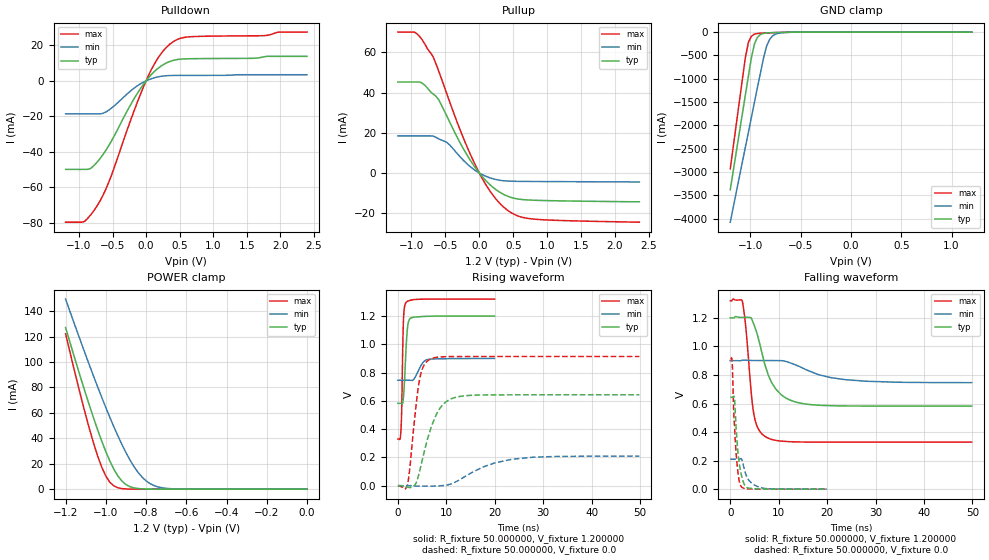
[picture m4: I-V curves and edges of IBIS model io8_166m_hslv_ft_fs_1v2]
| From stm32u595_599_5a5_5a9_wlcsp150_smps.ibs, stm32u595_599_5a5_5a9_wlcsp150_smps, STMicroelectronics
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|   Model io8_166m_hslv_ft_fs_1v2
[Model]  io8_166m_hslv_ft_fs_1v2
Model_type I/O
Polarity   Non-Inverting
Enable   Active-Low
Vinl =   0.360000V
Vinh =   0.840000V
Vmeas =  0.600000V
Cref =   50.000000pF
Rref =   100.000000M
Vref =   0.0V
C_comp   3.151700pF   3.087200pF   3.197900pF
[Temperature Range]   25.000000   0.140000k   -40.000000
[Pullup Reference]   1.200000V   0.900000V   1.320000V
[Pulldown Reference]   0.0V   0.0V   0.0V
[POWER Clamp Reference]   1.200000V   0.900000V   1.320000V
[GND Clamp Reference]   0.0V   0.0V   0.0V
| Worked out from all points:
|   slope of the pulldown table from 0 to 0.18 V, typ, clamps not added: 25.4 ohm
|   slope of the pullup table from 0 to 0.18 V, typ, clamps not added: 27.8 ohm
|   GND clamp passes 1 mA (typ) near -0.51 V on its own axis
|   POWER clamp passes 1 mA (typ) near -0.86 V on its own axis
|   rising waveform, R_fixture 50.000000, V_fixture 1.200000: 20-80 % time 569ps typ, 1.42ns min, 326ps max; typ from 0.582 V to 1.2 V
|   rising waveform, R_fixture 50.000000, V_fixture 0.0: 20-80 % time 3.44ns typ, 8.15ns min, 1.74ns max; typ from 0 V to 0.643 V
|   falling waveform, R_fixture 50.000000, V_fixture 1.200000: 20-80 % time 3.68ns typ, 8.13ns min, 1.62ns max; typ from 1.2 V to 0.582 V
|   falling waveform, R_fixture 50.000000, V_fixture 0.0: 20-80 % time 1.04ns typ, 1.73ns min, 833ps max; typ from 0.643 V to 0 V
[Pulldown]
|Voltage   I(typ)   I(min)   I(max)
-1.2V     -49.86mA   -18.57mA   -79.57mA
-920mV    -49.86mA   -18.57mA   -79.2mA
-840mV    -49.6mA    -18.57mA   -76.08mA
-720mV    -45.32mA   -18.57mA   -69.74mA
-560mV    -36.71mA   -16.58mA   -57.44mA
-200mV    -11.43mA   -4.74mA    -19.03mA
0V        10fA       -600fA     0A
160mV     6.477mA    2.075mA    11.78mA
360mV     10.99mA    2.99mA     20.81mA
480mV     12.07mA    3.054mA    23.53mA
640mV     12.43mA    3.075mA    24.76mA
2.4V      13.79mA    3.434mA    27.44mA
[Pullup]
|Voltage   I(typ)   I(min)   I(max)
-1.2V     45.31mA    18.46mA    70.13mA
-920mV    45.31mA    18.46mA    69.35mA
-840mV    44.69mA    18.46mA    66.15mA
-680mV    39.3mA     18.37mA    57.86mA
-600mV    36.53mA    16.99mA    50.82mA
-480mV    28.42mA    15.27mA    39.5mA
-280mV    14.84mA    7.944mA    21.22mA
-80mV     3.667mA    1.75mA     5.47mA
160mV     -5.889mA   -2.43mA    -9.115mA
400mV     -11.31mA   -3.958mA   -18.11mA
800mV     -13.54mA   -4.214mA   -22.92mA
2.36V     -14.3mA    -4.5mA     -24.47mA
[GND_clamp]
|Voltage   I(typ)   I(min)   I(max)
-1.2V     -3.379A    -4.076A    -2.932A
-1.05V    -1.35A     -2.47A     -550.7mA
-1.02V    -947.8mA   -2.149A    -221.5mA
-990mV    -552.4mA   -1.829A    -88.44mA
-960mV    -255.3mA   -1.51A     -44.87mA
-930mV    -111.8mA   -1.191A    -30.68mA
-870mV    -28.36mA   -564.6mA   -21.34mA
-840mV    -18.65mA   -309.5mA   -18.49mA
-810mV    -14.07mA   -161.6mA   -15.92mA
-780mV    -11.37mA   -83.33mA   -13.53mA
-600mV    -3.009mA   -4.322mA   -3.091mA
1.2V      0A         13.65nA    0A
[POWER_clamp]
|Voltage   I(typ)   I(min)   I(max)
-1.2V     127mA      149.4mA    122.2mA
-1.12V    84.97mA    114mA      70.27mA
-1.06V    55.51mA    88.42mA    35.67mA
-1.02V    37.63mA    72.04mA    17.17mA
-1V       29.51mA    64.13mA    10.3mA
-960mV    15.69mA    48.99mA    2.571mA
-900mV    3.624mA    28.77mA    182.8uA
-840mV    490.7uA    13.24mA    11.35uA
-800mV    116.8uA    6.532mA    1.77uA
-740mV    13.2uA     1.723mA    109.1nA
-620mV    167.4nA    79.36uA    0A
0V        0A         17.87nA    0A
[Ramp]
| variable   typ   min   max
dV/dt_r  0.38561/3.43218n   0.12545/8.14393n   0.54824/1.73724n
dV/dt_f  0.37085/3.67152n   92.35200m/8.14180n  0.59438/1.62007n
R_load = 50.000000
[Rising Waveform]
R_fixture= 50.000000
V_fixture= 1.200000
V_fixture_min= 0.900000
V_fixture_max= 1.320000
|time   V(typ)   V(min)   V(max)
0s        581.9mV    745.9mV    329.5mV
640.6ps   581.9mV    745.9mV    402mV
800.8ps   579.4mV    745.9mV    576.2mV
1.121ns   619.7mV    745.9mV    1.149V
1.321ns   718mV      745.9mV    1.257V
1.682ns   974mV      746mV      1.296V
2.122ns   1.15V      746mV      1.306V
2.843ns   1.188V     744.3mV    1.314V
6.126ns   1.198V     892.6mV    1.32V
19.94ns   1.2V       900mV      1.32V
[Rising Waveform]
R_fixture= 50.000000
V_fixture= 0.0
V_fixture_min= 0.0
V_fixture_max= 0.0
|time   V(typ)   V(min)   V(max)
0s        -5.803uV   240.9nV    -33.16uV
2.002ns   -9.17mV    -3.345uV   11.99mV
3.504ns   5.65mV     -2.808mV   493mV
4.404ns   92.41mV    -2.958mV   739.6mV
5.205ns   207.6mV    -2.965mV   839.8mV
6.406ns   363mV      -3.29mV    889.8mV
8.909ns   558.3mV    -280.5uV   911.1mV
12.51ns   629.6mV    37.95mV    913.7mV
23.52ns   642.7mV    187mV      913.9mV
49.85ns   642.9mV    209.3mV    913.9mV
[Falling Waveform]
R_fixture= 50.000000
V_fixture= 1.200000
V_fixture_min= 0.900000
V_fixture_max= 1.320000
|time   V(typ)   V(min)   V(max)
0s        1.2V       900mV      1.32V
2.503ns   1.203V     903.1mV    1.315V
3.203ns   1.203V     903.2mV    1.135V
4.805ns   1.16V      901.2mV    538.9mV
5.806ns   1.055V     901mV      421.4mV
7.307ns   856mV      901mV      366.3mV
10.41ns   664.7mV    900.5mV    337mV
15.12ns   598.6mV    845.4mV    330.2mV
23.62ns   582.9mV    767.4mV    329.4mV
49.85ns   581.9mV    745.9mV    329.5mV
[Falling Waveform]
R_fixture= 50.000000
V_fixture= 0.0
V_fixture_min= 0.0
V_fixture_max= 0.0
|time   V(typ)   V(min)   V(max)
0s        642.9mV    209.3mV    913.9mV
400.4ps   642.9mV    209.4mV    887mV
680.7ps   648mV      209.4mV    573.9mV
840.8ps   644mV      209.4mV    462.9mV
1.441ns   314.8mV    209.3mV    162.6mV
1.842ns   183.3mV    210.5mV    58.39mV
2.202ns   113.7mV    214.3mV    20.58mV
3.243ns   15.49mV    101.6mV    3.596mV
5.806ns   1.895mV    16.15mV    507.2uV
19.94ns   -5.803uV   240.9nV    -33.16uV
